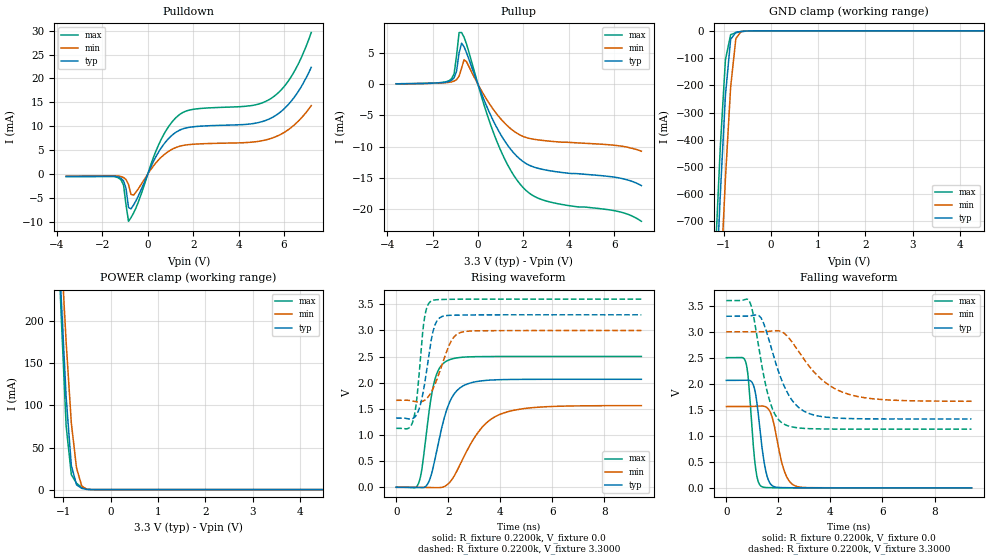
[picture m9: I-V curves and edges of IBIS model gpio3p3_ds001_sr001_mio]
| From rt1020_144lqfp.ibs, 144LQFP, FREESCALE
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[Model] gpio3p3_ds001_sr001_mio
|   Model gpio3p3_ds001_sr001_mio
| This model was characterised for following simulation conditions:
| External (pad) voltage:
|   - Typ: 3.3V,   - Min: 3.0V,   - Max: 3.6V
| Library cells for typ/min/max conditions are connected as defined below:
|  pad - External Pad
|  ipp_do - Core Input
|  ipp_obe - Output Buffer Enable
|  esd_boost - ovdd
|  ipp_dse0 - vddi
|  ipp_dse1 - vssi
|  ipp_dse2 - vssi
|  ipp_fsel0 - vddi
|  ipp_fsel1 - vssi
|  ipp_ina - ipp_ina
|  ipp_ind - ipp_ind
|  ipp_pwr_stable - vddi
|  ipp_sre - vssi
|  ovdd - ovdd
|  ovss - ovss
|  vddi - vddi
|  vssi - vssi
| All other pins connected to ground
Model_type I/O
Polarity   Non-Inverting
Enable   Active-High
Vinl =   0.9900V
Vinh =   2.3100V
Vmeas =  1.6500V
Cref =   0.0F
Rref =   0.2200k
Vref =   1.6500V
C_comp   1.2178pF   1.1833pF   1.2636pF
|C_comp_pullup   0.6042pF   0.6189pF   0.5908pF
|C_comp_pulldown   0.5474pF   0.5788pF   0.5258pF
[Model Spec]
| variable   typ   min   max
Vinh   2.3100V   2.1000V   2.5200V
Vinl   0.9900V   0.9000V   1.0800V
S_overshoot_high   3.3000V   3.0000V   3.6000V
S_overshoot_low   0.0V   0.0V   0.0V
Vmeas   1.6500V   1.5000V   1.8000V
Vref   1.6500V   1.5000V   1.8000V
Cref   0.0F   0.0F   0.0F
Rref   0.2200k   0.2200k   0.2200k
[Temperature Range]   25.0000   0.1050k   -20.0000
[Voltage Range]   3.3000V   3.0000V   3.6000V
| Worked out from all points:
|   slope of the pulldown table from 0 to 0.495 V, typ, clamps not added: 104 ohm
|   slope of the pullup table from 0 to 0.495 V, typ, clamps not added: 112 ohm
|   GND clamp passes 1 mA (typ) near -0.54 V on its own axis
|   POWER clamp passes 1 mA (typ) near -0.57 V on its own axis
|   rising waveform, R_fixture 0.2200k, V_fixture 0.0: 20-80 % time 640ps typ, 1.18ns min, 426ps max; typ from 0 V to 2.07 V
|   rising waveform, R_fixture 0.2200k, V_fixture 3.3000: 20-80 % time 385ps typ, 592ps min, 275ps max; typ from 1.32 V to 3.3 V
|   falling waveform, R_fixture 0.2200k, V_fixture 0.0: 20-80 % time 310ps typ, 419ps min, 233ps max; typ from 2.07 V to 0 V
|   falling waveform, R_fixture 0.2200k, V_fixture 3.3000: 20-80 % time 875ps typ, 1.46ns min, 582ps max; typ from 3.3 V to 1.32 V
[Pulldown]
|Voltage   I(typ)   I(min)   I(max)
-3.6V     -510uA     -430uA     -540uA
-1.29V    -647uA     -417uA     -827uA
-1.07V    -1.427mA   -731.3uA   -2.281mA
-960mV    -2.986mA   -1.137mA   -6.485mA
-850mV    -7mA       -2.186mA   -9.891mA
-630mV    -6.507mA   -4.426mA   -8.193mA
470mV     4.567mA    2.939mA    6.048mA
1.24V     8.736mA    5.546mA    11.79mA
1.9V      9.822mA    6.191mA    13.44mA
5.42V     11.68mA    7.43mA     15.78mA
6.3V      15.14mA    9.67mA     20.23mA
7.2V      22.31mA    14.31mA    29.59mA
[Pullup]
|Voltage   I(typ)   I(min)   I(max)
-3.6V     80uA       60uA       70uA
-1.16V    634uA      374uA      887uA
-1.05V    1.031mA    497uA      1.681mA
-940mV    2.112mA    740uA      4.609mA
-830mV    5.029mA    1.286mA    8.268mA
-720mV    6.574mA    2.584mA    8.272mA
-610mV    5.992mA    3.932mA    7.525mA
-500mV    5.025mA    3.584mA    6.406mA
820mV     -6.857mA   -4.721mA   -9.018mA
2.03V     -12.48mA   -8.409mA   -16.69mA
3.02V     -13.75mA   -9.063mA   -18.7mA
7.2V      -16.22mA   -10.72mA   -21.94mA
[GND_clamp]
|Voltage   I(typ)   I(min)   I(max)
-3.6V     -10.99A    -11.14A    -10.93A
-1.18V    -1.033A    -1.378A    -850.8mA
-1.07V    -607mA     -947.1mA   -431.4mA
-960mV    -236.8mA   -543mA     -106.4mA
-850mV    -31.63mA   -206.7mA   -14.18mA
-740mV    -5.424mA   -29mA      -7.092mA
-630mV    -2.275mA   -2.653mA   -3.283mA
-410mV    -62.05uA   -83.52uA   -82.05uA
7.2V      0A         0A         0A
[POWER_clamp]
|Voltage   I(typ)   I(min)   I(max)
-3.6V     3.491A     3.319A     3.949A
-1.16V    368.2mA    410.8mA    372.9mA
-1.05V    234.5mA    290.2mA    214.3mA
-940mV    110.2mA    175.6mA    75.85mA
-830mV    28.53mA    79.02mA    17.73mA
-720mV    5.671mA    25.66mA    7.515mA
-610mV    1.49mA     4.301mA    2.636mA
-500mV    198.2uA    300.8uA    424.4uA
-390mV    9.667uA    18.86uA    16.14uA
7.2V      0A         0A         0A
[Ramp]
| variable   typ   min   max
dV/dt_r  1.2397/0.6401n   0.9377/1.1757n   1.5016/0.4265n
dV/dt_f  1.1856/0.8752n   0.8012/1.4587n   1.4829/0.5817n
R_load = 0.2200k
[Rising Waveform]
R_fixture= 0.2200k
V_fixture= 0.0
V_fixture_min= 0.0
V_fixture_max= 0.0
|time   V(typ)   V(min)   V(max)
0s        16.92nV    15.3nV     179.1nV
860.6ps   -6.867mV   -208.6uV   78.47mV
993.9ps   -9.29mV    -1.259mV   372.3mV
1.191ns   51.63mV    -3.233mV   1.175V
1.45ns    449mV      -6.086mV   1.992V
1.961ns   1.513V     49.01mV    2.422V
2.556ns   1.936V     538.9mV    2.489V
3.211ns   2.033V     1.095V     2.501V
3.944ns   2.058V     1.386V     2.502V
9.42ns    2.066V     1.563V     2.503V
[Rising Waveform]
R_fixture= 0.2200k
V_fixture= 3.3000
V_fixture_min= 3.0000
V_fixture_max= 3.6000
|time   V(typ)   V(min)   V(max)
0s        1.324V     1.664V     1.129V
484.3ps   1.308V     1.663V     1.133V
666.1ps   1.324V     1.647V     1.305V
805ps     1.408V     1.634V     1.756V
1.072ns   1.919V     1.659V     3.188V
1.364ns   2.865V     1.837V     3.568V
1.654ns   3.236V     2.187V     3.591V
2.097ns   3.291V     2.784V     3.597V
2.516ns   3.296V     2.968V     3.599V
9.42ns    3.3V       3V         3.6V
[Falling Waveform]
R_fixture= 0.2200k
V_fixture= 0.0
V_fixture_min= 0.0
V_fixture_max= 0.0
|time   V(typ)   V(min)   V(max)
0s        2.066V     1.563V     2.503V
757.7ps   2.071V     1.564V     2.395V
858.5ps   2.071V     1.564V     2.026V
1.131ns   1.787V     1.567V     350.9mV
1.361ns   815.9mV    1.573V     23.34mV
1.542ns   268.6mV    1.55V      5.866mV
1.709ns   67.39mV    1.433V     3.676mV
2.209ns   3.835mV    351.2mV    1.514mV
2.648ns   2.046mV    37.5mV     684.8uV
9.42ns    804.1nV    5.147uV    482.8nV
[Falling Waveform]
R_fixture= 0.2200k
V_fixture= 3.3000
V_fixture_min= 3.0000
V_fixture_max= 3.6000
|time   V(typ)   V(min)   V(max)
0s        3.3V       3V         3.6V
908.7ps   3.305V     3V         3.564V
1.312ns   3.281V     3V         2.501V
1.619ns   2.878V     3.009V     1.753V
1.866ns   2.451V     3.021V     1.415V
2.241ns   1.936V     2.965V     1.218V
3.077ns   1.45V      2.408V     1.141V
3.762ns   1.363V     2.042V     1.131V
4.617ns   1.334V     1.812V     1.129V
9.42ns    1.324V     1.665V     1.129V
